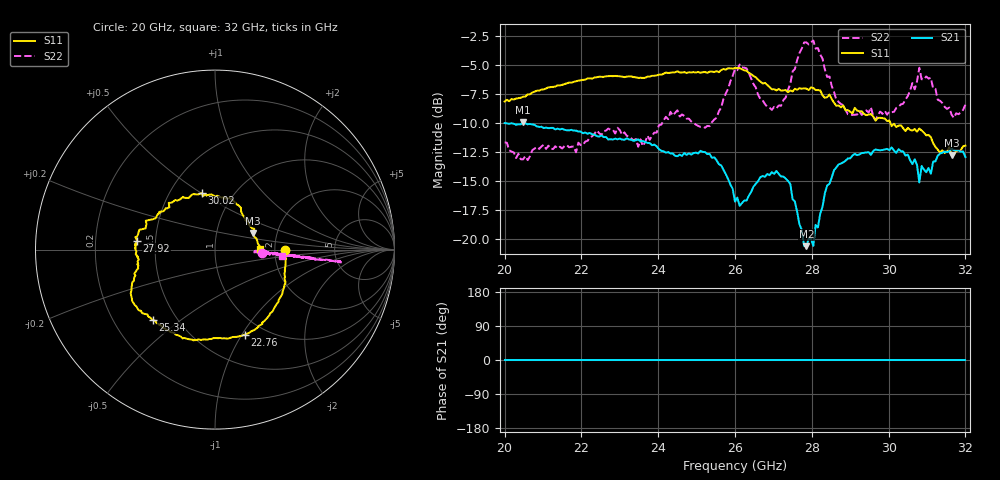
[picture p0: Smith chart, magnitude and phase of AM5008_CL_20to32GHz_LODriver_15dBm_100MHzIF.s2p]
!Keysight Technologies,N5245B,MY58422270,A.16.20.02
!Mixer S2P File: Scalar Mixer Measurement
!Calibration State: On
!Parameters: Stimulus Freq, S11, SC21, SC12, S22
# Hz  S  DB  R  50.0
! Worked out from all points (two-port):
!   201 points, 20 GHz to 32 GHz, reference 50 ohm
!   highest |S21| = -9.94 dB at 20.48 GHz (marker M1); lowest = -20.6 dB at 27.86 GHz (marker M2)
!   |S21| within 3 dB of the highest: start of sweep to 25.39 GHz; 29.03 GHz to 30.52 GHz (1.493 GHz wide, 5.01 % of centre)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
!   lowest |S11| = -12.8 dB at 31.64 GHz (marker M3), VSWR 1.59, Z = 74.7 + j14.6 ohm
!   |S11| at or under -10 dB: 30.04 GHz to end of sweep
!   |S22| runs from -13.2 to -2.9 dB; largest |S21 - S12| = 0.32
!   S11 on the Smith chart (normalised r, x): 20 GHz: 2.28, -0.00; 22.76 GHz: 0.82, -1.03; 25.34 GHz: 0.37, -0.40; 27.92 GHz: 0.39, +0.05; 30.02 GHz: 0.72, +0.50; 32 GHz: 1.67, +0.02
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2e10  -8.17 -0.1  -10.03 0.0  -200.00 90.0  -11.70 -3.9
2.048e10  -7.77 -17.8  -9.94 0.0  -200.00 90.0  -13.16 -3.3
2.204e10  -6.31 -55.5  -10.91 0.0  -200.00 90.0  -11.94 -3.7
2.276e10  -5.98 -70.5  -11.42 0.0  -200.00 90.0  -10.61 -6.2
2.348e10  -6.14 -86.7  -11.43 0.0  -200.00 90.0  -12.07 -3.1
2.402e10  -5.86 -98.8  -12.29 0.0  -200.00 90.0  -10.22 -3.9
2.45e10  -5.57 -110.1  -12.89 0.0  -200.00 90.0  -8.94 -4.6
2.534e10  -5.61 -131.6  -12.69 0.0  -200.00 90.0  -10.30 -3.5
2.6e10  -5.30 -145.4  -16.79 0.0  -200.00 90.0  -5.38 -5.2
2.72e10  -7.25 -169.8  -14.63 0.0  -200.00 90.0  -8.54 -4.1
2.744e10  -7.23 -174.8  -15.27 0.0  -200.00 90.0  -6.66 -4.8
2.786e10  -7.07 177.0  -20.63 0.0  -200.00 90.0  -3.09 -5.3
2.792e10  -7.19 173.3  -19.97 0.0  -200.00 90.0  -3.26 -5.5
2.804e10  -7.01 171.7  -20.61 0.0  -200.00 90.0  -2.92 -5.8
2.858e10  -8.28 154.0  -14.09 0.0  -200.00 90.0  -7.37 -4.7
2.894e10  -8.91 139.9  -13.08 0.0  -200.00 90.0  -9.27 -3.7
3.002e10  -9.81 103.2  -12.37 0.0  -200.00 90.0  -9.05 -3.9
3.068e10  -10.54 79.4  -13.15 0.0  -200.00 90.0  -7.13 -4.2
3.08e10  -10.51 73.7  -15.14 0.0  -200.00 90.0  -5.27 -4.8
3.086e10  -10.67 70.6  -13.72 0.0  -200.00 90.0  -6.26 -5.4
3.164e10  -12.82 23.8  -12.23 0.0  -200.00 90.0  -9.31 -3.8
3.2e10  -11.98 1.2  -12.96 0.0  -200.00 90.0  -8.46 -5.8
